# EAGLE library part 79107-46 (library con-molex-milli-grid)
RECEPTACAL
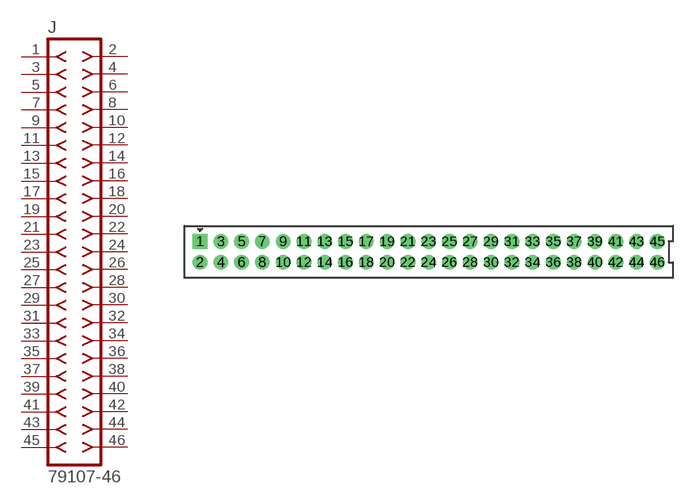
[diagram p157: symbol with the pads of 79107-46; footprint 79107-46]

Designator prefix J

## 79107-46  [79107-46]
1  1  pas
2  2  pas
3  3  pas
4  4  pas
5  5  pas
6  6  pas
7  7  pas
8  8  pas
9  9  pas
10  10  pas
11  11  pas
12  12  pas
13  13  pas
14  14  pas
15  15  pas
16  16  pas
17  17  pas
18  18  pas
19  19  pas
20  20  pas
21  21  pas
22  22  pas
23  23  pas
24  24  pas
25  25  pas
26  26  pas
27  27  pas
28  28  pas
29  29  pas
30  30  pas
31  31  pas
32  32  pas
33  33  pas
34  34  pas
35  35  pas
36  36  pas
37  37  pas
38  38  pas
39  39  pas
40  40  pas
41  41  pas
42  42  pas
43  43  pas
44  44  pas
45  45  pas
46  46  pas

## Footprint 79107-46 (pad centres in mm)
RECEPTACAL Dual Row, Vertical, Through-Hole
drill 0.914 square: 1 -22,1
drill 0.914: 2 -22,-1; 3 -20,1; 4 -20,-1; 5 -18,1; 6 -18,-1; 7 -16,1; 8 -16,-1; 9 -14,1; 10 -14,-1; 11 -12,1; 12 -12,-1; 13 -10,1; 14 -10,-1; 15 -8,1; 16 -8,-1; 17 -6,1; 18 -6,-1; 19 -4,1; 20 -4,-1; 21 -2,1; 22 -2,-1; 23 0,1; 24 0,-1; 25 2,1; 26 2,-1; 27 4,1; 28 4,-1; 29 6,1; 30 6,-1; 31 8,1; 32 8,-1; 33 10,1; 34 10,-1; 35 12,1; 36 12,-1; 37 14,1; 38 14,-1; 39 16,1; 40 16,-1; 41 18,1; 42 18,-1; 43 20,1; 44 20,-1; 45 22,1; 46 22,-1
